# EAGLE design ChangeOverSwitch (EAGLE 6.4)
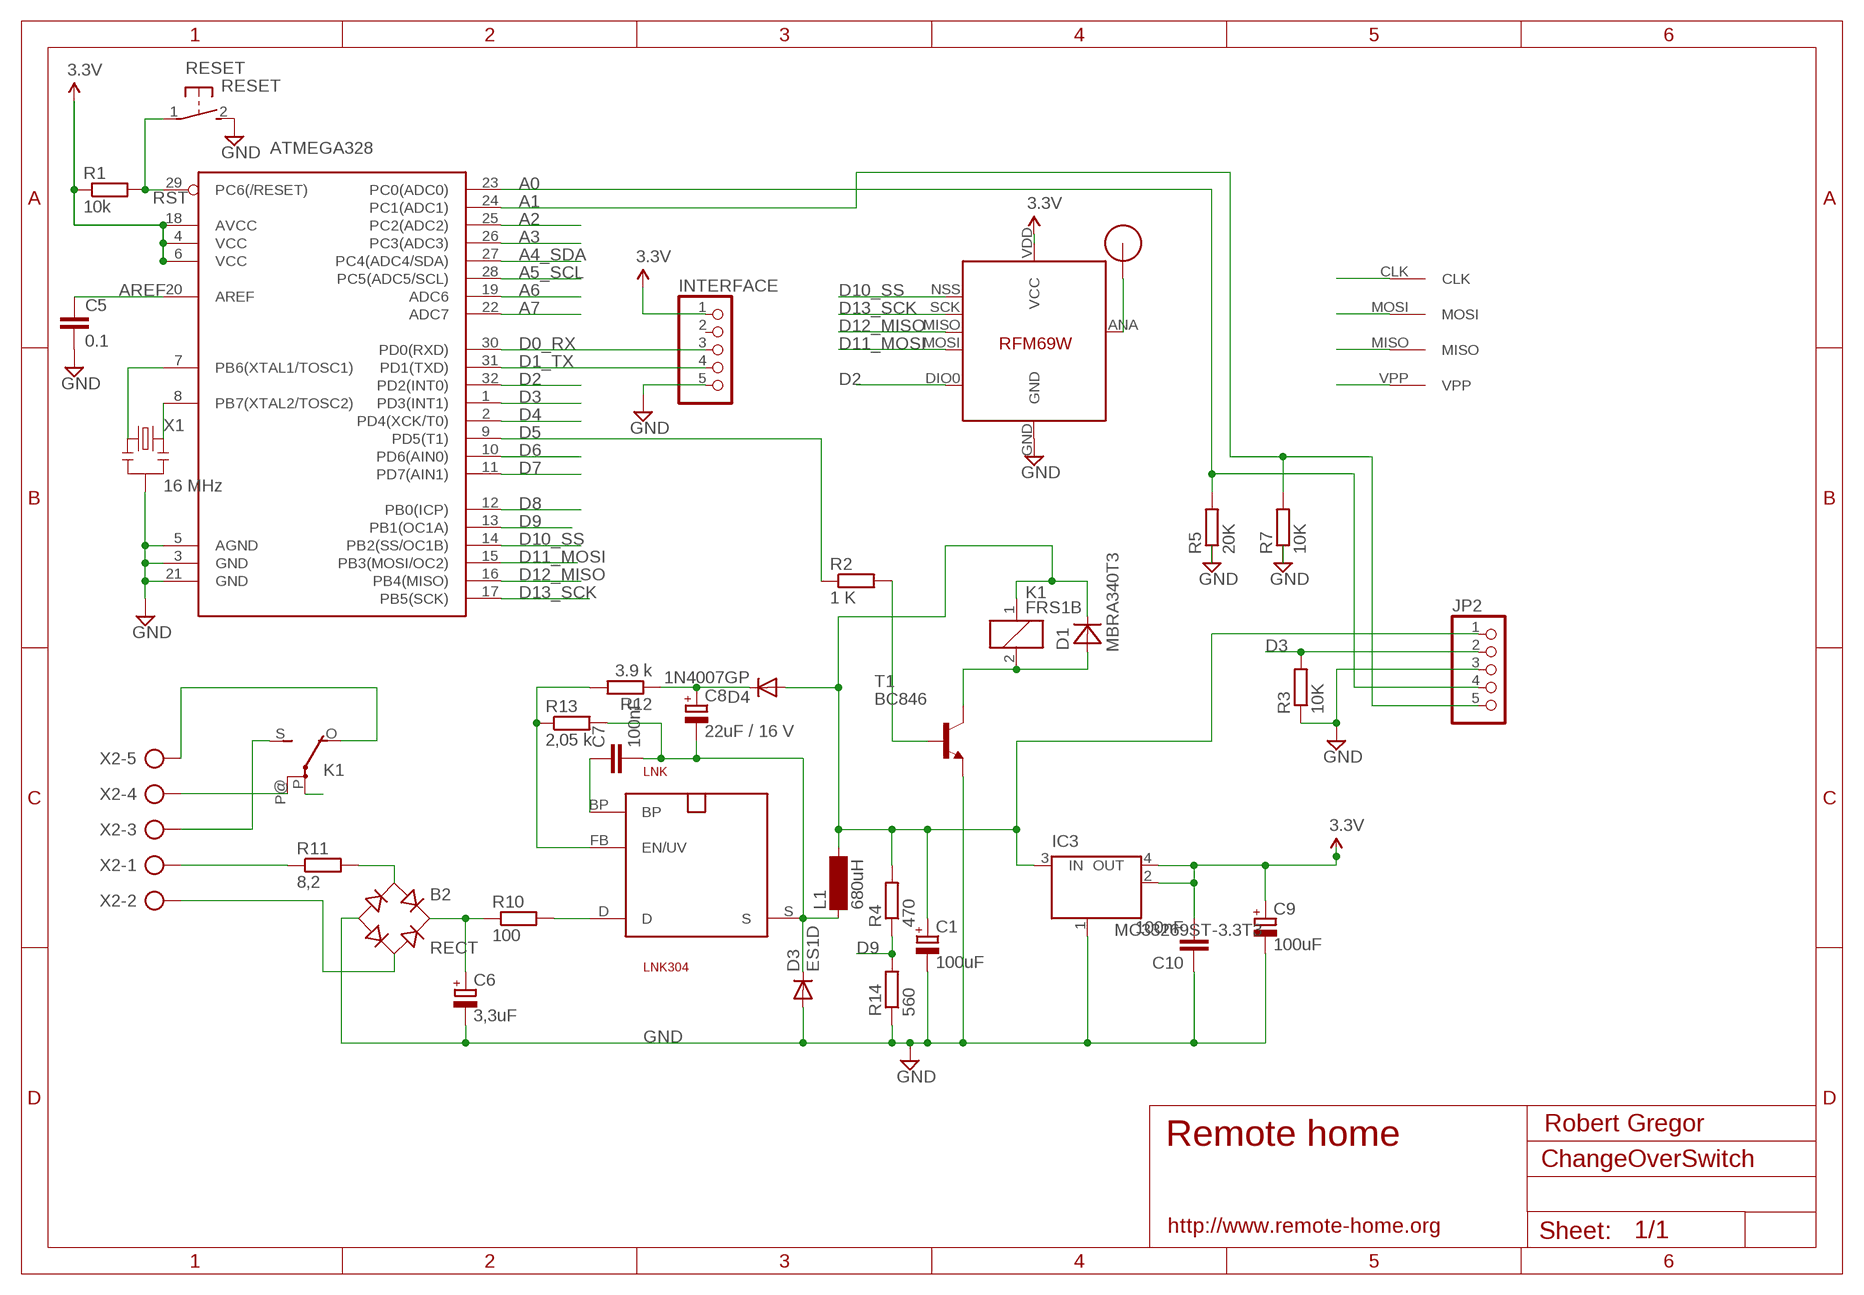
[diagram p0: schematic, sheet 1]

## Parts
ATMEGA328  ATMega-328  ATMEGA168/328TQFP32  [TQFP32-08]
B2  RECT  RECTIFIER-S40  [TO-269AA]
C1  100uF  CPOL-EUSMCB  [SMC_B]
C5  0.1  C-EUC2012  [C2012]
C6  3,3uF  CPOL-EUE5-10.5  [E5-10,5]
C7  100nF  C-EUC2012  [C2012]
C8  22uF / 16 V  CPOL-EUSMCC  [SMC_C]
C9  100uF  CPOL-EUSMCB  [SMC_B]
C10  100nF  C-EUC2012  [C2012]
D1  MBRA340T3  [SMA]
D3  ES1D  DIODE-DO214AC  [DO214AC]
D4  1N4007GP  DIODE-DO214AA  [DO214AA]
IC3  MC33269ST-3.3T3  [SOT223]
INTERFACE  PINHD-1X05_2.54-S  [1X05-S]
JP2  PINHD-1X05_2.00  [1X05M]
K1  FRS1B  [FRS1B]
L1  680uH  BS11  [BS11]
LNK  LNK304  SO-8C  [SO-8C]
R1  10k  R-EU_R2012  [R2012]
R2  1 K  R-EU_M2012  [M2012]
R3  10K  R-EU_M2012  [M2012]
R4  470  R-EU_M2012  [M2012]
R5  20K  R-EU_M2012  [M2012]
R7  10K  R-EU_M2012  [M2012]
R10  100  R-EU_R2512W  [R2512W]
R11  8,2  R-EU_0411/12  [0411/12]
R12  3.9 k  R-EU_M2012  [M2012]
R13  2,05 k  R-EU_M2012  [M2012]
R14  560  R-EU_M2012  [M2012]
RESET  RESET  DTSM-3  [DTSM-3]
RFM69  RFM69  [RFM69W-MINPADS]
T1  BC846  [SOT23]
U$1  RFM12B_ANTENNA  [RFM12B-ANTENNA]
U$2  AVRHEADERDIP  [AVRHEADER]
X1  16 MHz  RESONATORSMD  [RESONATOR-SMD]
X2  AK500/5  [AK500/5]

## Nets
5V: C1.+ D1.C D4.A IC3.3(IN) JP2.1 K1.1 L1.2 R4.2
A0: ATMEGA328.23(PC0(ADC0)) JP2.4 R5.2
A1: ATMEGA328.24(PC1(ADC1)) JP2.5 R7.2
A2: ATMEGA328.25(PC2(ADC2))
A3: ATMEGA328.26(PC3(ADC3))
A4_SDA: ATMEGA328.27(PC4(ADC4/SDA))
A5_SCL: ATMEGA328.28(PC5(ADC5/SCL))
A6: ATMEGA328.19(ADC6)
A7: ATMEGA328.22(ADC7)
AREF: ATMEGA328.20(AREF) C5.1
D0_RX: ATMEGA328.30(PD0(RXD)) INTERFACE.3
D1_TX: ATMEGA328.31(PD1(TXD)) INTERFACE.4
D2: ATMEGA328.32(PD2(INT0)) RFM69.DIO0
D3: ATMEGA328.1(PD3(INT1)) JP2.2 R3.2
D4: ATMEGA328.2(PD4(XCK/T0))
D5: ATMEGA328.9(PD5(T1)) R2.1
D6: ATMEGA328.10(PD6(AIN0))
D7: ATMEGA328.11(PD7(AIN1))
D8: ATMEGA328.12(PB0(ICP))
D9: ATMEGA328.13(PB1(OC1A)) R4.1 R14.2
D10_SS: ATMEGA328.14(PB2(SS/OC1B)) RFM69.NSS(SEL)
D11_MOSI: ATMEGA328.15(PB3(MOSI/OC2)) RFM69.MOSI U$2.MOSI
D12_MISO: ATMEGA328.16(PB4(MISO)) RFM69.MISO U$2.MISO
D13_SCK: ATMEGA328.17(PB5(SCK)) RFM69.SCK U$2.CLK
FB: LNK.FB(EN/UV) R12.2 R13.1
GND [power]: ATMEGA328.3(GND) ATMEGA328.5(AGND) ATMEGA328.21(GND) B2.- C1.- C5.2 C6.- C9.- C10.1 D3.A IC3.1(GND/ADJ) INTERFACE.5 JP2.3 R3.1 R5.1 R7.1 R14.1 RESET.2 RFM69.GND T1.2(E) X1.2
N$1: ATMEGA328.7(PB6(XTAL1/TOSC1)) X1.1
N$2: R2.2 T1.1(B)
N$3: RFM69.ANA(ANT) U$1.P$1
N$5: D1.A K1.2 T1.3(C)
N$6 [220V]: K1.P(2:P)
N$7 [220V]: R11.1 X2.1
N$8 [220V]: K1.P@(2:P) X2.4
N$9 [220V]: B2.AC2 X2.2
N$10: C7.2 C8.- D3.C L1.1 LNK.S R13.2
N$11 [220V]: K1.S(2:S) X2.3
N$12 [220V]: K1.O(2:O) X2.5
N$13 [220V]: LNK.D R10.2
N$14 [220V]: B2.+ C6.+ R10.1
N$15 [220V]: B2.AC1 R11.2
N$18: C7.1 LNK.BP
N$20: C8.+ D4.C R12.1
N$21: ATMEGA328.8(PB7(XTAL2/TOSC2)) X1.3
RST: ATMEGA328.29(PC6(/RESET)) R1.2 RESET.1 U$2.VPP
VCC: ATMEGA328.4(VCC) ATMEGA328.6(VCC) ATMEGA328.18(AVCC) C9.+ C10.2 IC3.2(OUT) IC3.4(OUT) INTERFACE.1 R1.1 RFM69.VDD(VCC) ; supply symbol labelled 3.3V
Unconnected: INTERFACE.2

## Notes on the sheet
- Robert Gregor
- Remote home
- http://www.remote-home.org

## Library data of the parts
ATMEGA328 = LowPowerLab:ATMEGA168/328: Atmel 32-pin 8-bit micro, 16k flash.
B2 = rectifier:RECTIFIER-: Rectifier
C1 C6 C8 C9 = resistor:CPOL-EU: POLARIZED CAPACITOR, European symbol
C5 C7 C10 = resistor:C-EU: CAPACITOR, European symbol
D1 = diode:MBRA340T3: Surface Mount Schottky Power Rectifier
D3 D4 = diode:DIODE-: DIODE
IC3 = linear:MC33269ST*: Adjustable Output Low Dropout Voltage Regulator 800 mA Source: http://www.onsemi.com/pub/Collateral/MC33269-D.PDF
INTERFACE JP2 = pinhead-2:PINHD-1X05: PIN HEADER
K1 = relay:FRS1B: RELAY 1 x switch, same as V23101-D6-A201, Siemens; OC_FARNELL: unknown; OC_NEWARK: unknown
L1 = inductor-neosid:BS: INDUCTOR; OC_FARNELL: unknown; OC_NEWARK: unknown
LNK = powerint:SO-8C: 700V MOSFET für Schaltnetz-Trafos. Pin 3 fehlt. SMD
R1-R5 R7 R10-R14 = resistor:R-EU_: RESISTOR, European symbol
RESET = switch-tact:DTSM-3
RFM69 = LowPowerLab:RFM69
T1 = transistor:BC846: NPN TRANSISTOR
U$1 = LowPowerLab:RFM12B_ANTENNA
U$2 = RemoteHome:AVRHEADER
X1 = SparkFun:RESONATOR: Resonator Small SMD resonator. This is the itty bitty 10/20MHz resonators with built in caps. CSTCE10M0G55 and CSTCE20M0V53. Footprint has been reviewed closely but hasn't been tested yet.
X2 = con-ptr500:AK500/5: CONNECTOR; OC_FARNELL: unknown; OC_NEWARK: unknown

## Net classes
1 power: width 0.381 mm, clearance 0.254 mm
2 220V: width 0.381 mm, clearance 0.508 mm

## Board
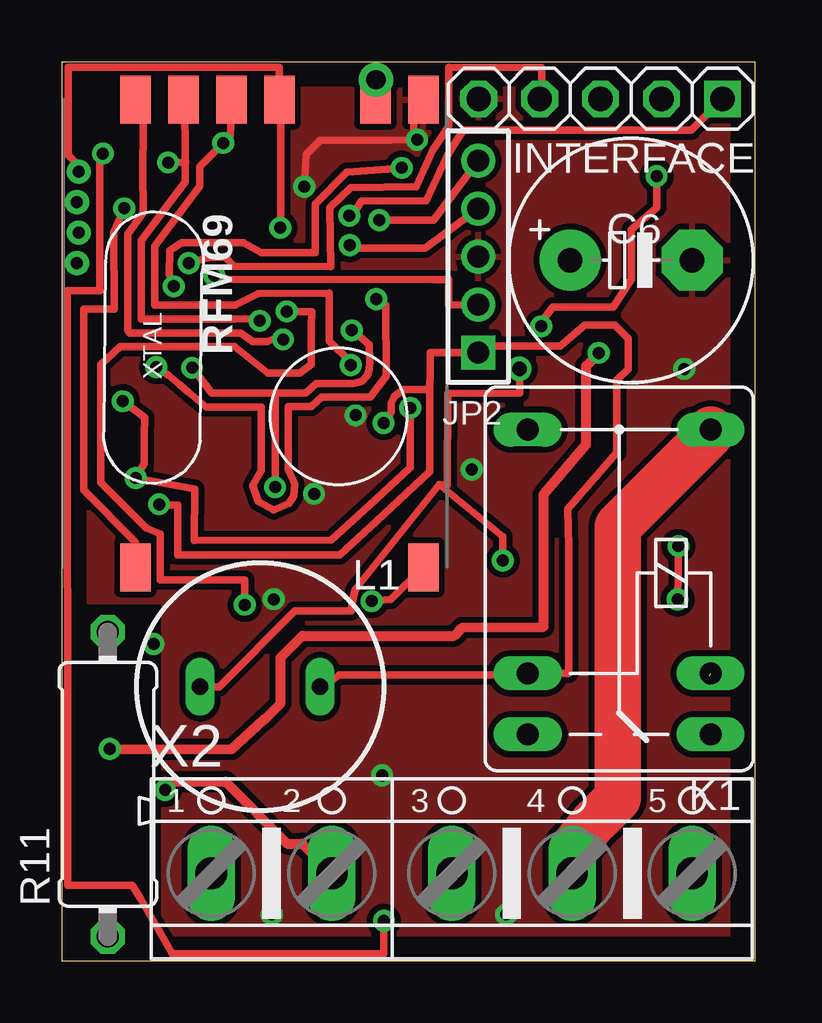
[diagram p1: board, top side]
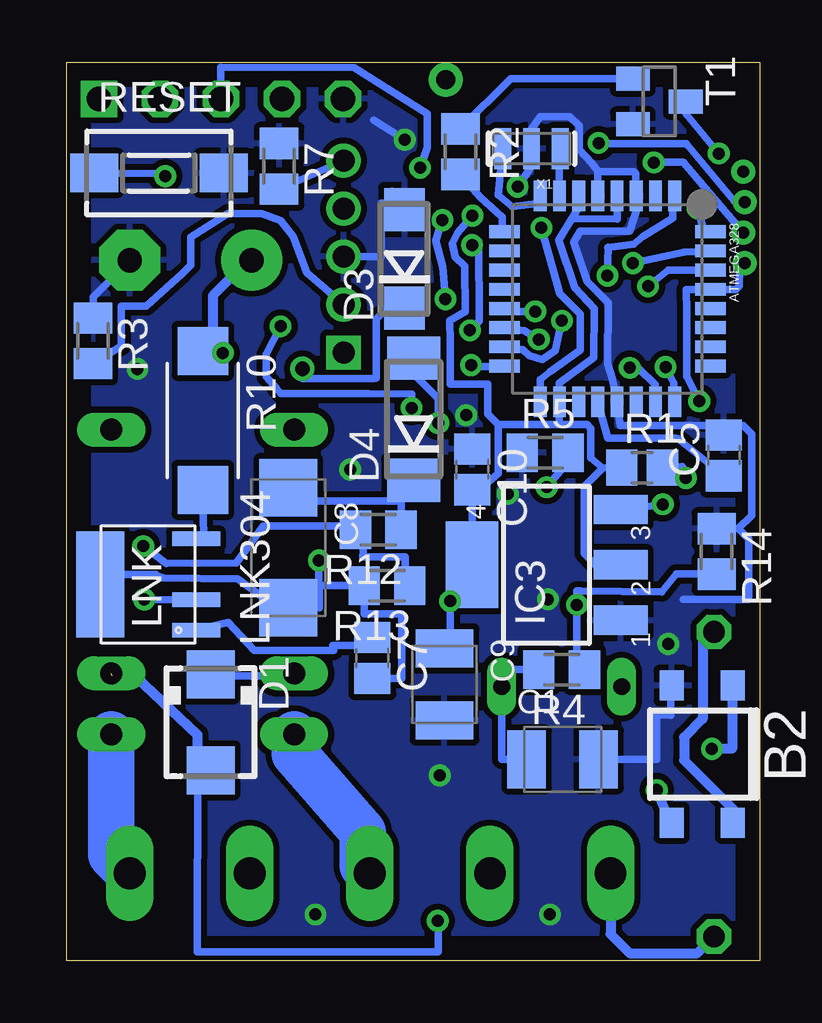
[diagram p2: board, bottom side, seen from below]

Size 28.88 x 37.45 mm. Coordinates in mm from the lower left corner, seen from the top.
Outline: 0,0 28.88,0 28.88,37.45 0,37.45 0,0
Copper layers (1*16): Top 0.035mm / dielectric 1.5mm / Bottom 0.035mm
Design rules "default": minimum track width 10mil, minimum drill 24mil, track to track 8mil, track to pad 8mil, pad to pad 8mil, via to via 8mil, smd to smd 8mil, copper to edge 40mil, drill to drill 8mil, minimum pad ring 10mil, minimum via ring 8mil, stop-mask expansion 4mil, vias tented up to drill 0mil, thermal gap 10mil

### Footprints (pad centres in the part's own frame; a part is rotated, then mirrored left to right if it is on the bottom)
TQFP32-08 = smd 1.27 x 0.533: 1 -4.293,2.8; 2 -4.293,2; 3 -4.293,1.2; 4 -4.293,0.4; 5 -4.293,-0.4; 6 -4.293,-1.2; 7 -4.293,-2; 8 -4.293,-2.8; 17 4.293,-2.8; 18 4.293,-2; 19 4.293,-1.2; 20 4.293,-0.4; 21 4.293,0.4; 22 4.293,1.2; 23 4.293,2; 24 4.293,2.8 | smd 0.533 x 1.27: 9 -2.8,-4.293; 10 -2,-4.293; 11 -1.2,-4.293; 12 -0.4,-4.293; 13 0.4,-4.293; 14 1.2,-4.293; 15 2,-4.293; 16 2.8,-4.293; 25 2.8,4.293; 26 2,4.293; 27 1.2,4.293; 28 0.4,4.293; 29 -0.4,4.293; 30 -1.2,4.293; 31 -2,4.293; 32 -2.8,4.293
TO-269AA = smd 1 x 1.25: + -1.28,-2.855; - 1.28,-2.855; AC1 -1.28,2.855; AC2 1.28,2.855
SMC_B = smd 1.6 x 2.4: + -1.5,0; - 1.5,0
C2012 = smd 1.3 x 1.5: 1 -0.85,0; 2 0.85,0
E5-10,5 = drill 1.016 pad 2.54: + -2.54,0 | drill 1.016 pad 2.54 octagon: - 2.54,0
SMC_C = smd 2.4 x 2.4: + -2.5,0; - 2.5,0
SMA = smd 2 x 2: A 2,0; C -2,0
DO214AC = smd 1.8 x 1.7: A 2.05,0; C -2.05,0
DO214AA = smd 1.8 x 2.2: A 2.55,0; C -2.55,0
SOT223 = smd 1.219 x 2.235: 1 -2.311,-3.099; 2 0,-3.099; 3 2.311,-3.099 | smd 3.6 x 2.2: 4 0,3.099
1X05-S = drill 1.016 square: 1 -5.08,0 | drill 1.016 octagon: 2 -2.54,0; 3 0,0; 4 2.54,0; 5 5.08,0
1X05M = drill 0.914 square: 1 -4,0 | drill 0.914: 2 -2,0; 3 0,0; 4 2,0; 5 4,0
FRS1B = drill 0.914 long: 1 0,3.81; 2 0,-3.81; O -2.54,-3.81; P 10.16,3.81; P@ 10.16,-3.81; S -2.54,3.81
BS11 = drill 0.7 long: 1 -2.5,0; 2 2.5,0
SO-8C = smd 0.6 x 2: BP -1.905,-2; D 1.905,-2; FB -0.635,-2 | smd 4.41 x 2: S 0,2
R2012 = smd 1.3 x 1.5: 1 -0.85,0; 2 0.85,0
M2012 = smd 1.3 x 1.6: 1 -0.95,0; 2 0.95,0
R2512W = smd 2 x 2.1: 1 -2.896,0; 2 2.896,0
0411/12 = drill 0.914 octagon: 1 -6.35,0; 2 6.35,0
DTSM-3 = smd 2 x 1.6: 1 -2.7,0; 2 2.7,0
RFM69W-MINPADS = smd 2 x 1.27: ANA 8,-5; DIO0 -11.5,5; GND 8,-7; MISO 8,1; MOSI 8,3; NSS 8,5; SCK 8,-1; VDD -11.5,-7
SOT23 = smd 1 x 1.4: 1 -0.95,-1.1; 2 0.95,-1.1; 3 0,1.1
RFM12B-ANTENNA = drill 0.8 pad 1.422: P$1 0,0
AVRHEADER = drill 0.5: CLK 2.54,0; MISO 1.27,0.07; MOSI 0,0; VPP -1.27,0.072
RESONATOR-SMD = smd 0.7 x 1.7: 1 -1.2,0; 2 0,0; 3 1.2,0
AK500/5 = drill 1.321 long: 1 -10.033,0; 2 -5.004,0; 3 0,0; 4 5.004,0; 5 10.008,0

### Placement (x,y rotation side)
ATMEGA328  6.35,27.59 270 bottom
B2  2.4,8.62 180 bottom
C1  8.22,8.4 0 bottom
C5  1.5,21.07 90 bottom
C6  23.71,29.21 0 top
C7  16.15,12.63 270 bottom
C8  19.65,17.22 270 bottom
C9  13.14,11.52 270 bottom
C10  11.98,20.49 270 bottom
D1  22.89,9.95 270 bottom
D3  14.8,29.26 90 bottom
D4  14.42,22.58 90 bottom
IC3  8.89,16.51 90 bottom
INTERFACE  22.45,35.94 180 top
JP2  17.34,29.36 90 top
K1  23.22,11.99 90 top
L1  8.26,11.43 0 top
LNK  25.49,15.69 90 bottom
R1  4.91,20.57 0 bottom
R2  12.47,33.74 90 bottom
R3  27.79,25.85 270 bottom
R4  8.26,12.14 180 bottom
R5  8.94,21.18 0 bottom
R7  20.03,33.13 270 bottom
R10  23.21,22.53 270 bottom
R11  1.91,7.36 90 top
R12  15.9,17.98 180 bottom
R13  15.53,15.64 180 bottom
R14  1.8,17.07 270 bottom
RESET  25.04,32.85 0 bottom
RFM69  8.06,27.91 90 top
T1  4.19,35.83 270 bottom
U$1  13.08,36.73 0 top
U$2  0.69,30.36 90 top
X1  9.51,33.86 180 bottom
X2  16.25,3.65 0 top

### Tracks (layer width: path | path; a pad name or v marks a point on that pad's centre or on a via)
5V  (via drill 0.5)
  Top 0.305: L1.2 10.88,11.43 10.89,11.44 10.89,11.38 11.56,11.92 18.64,11.93 18.87,11.92 K1.1 19.68,11.97 21.12,11.97 21.12,17.23 21.08,18.85 23.12,21.19 23.12,24.21 23.59,24.68 23.59,25.95 23.02,26.51 21.78,26.51 20.76,25.62 17.73,25.62 JP2.1 16.34,25.37 15.9,25.36 15.35,25.36 15.35,24.29 15.33,24.14 | 15.33,24.14 15.31,20.39 13.09,18.31 11.56,16.91 4.82,16.91 4.82,17.62 4.82,19.01 4.4,19.01 v4.04,19.03 | v13.4,22.42 13.73,22.88 13.72,23.26 13.85,23.53 14.21,23.81 15.33,23.81 15.33,24.14
  Bottom 0.305: D1.C 22.82,11.88 19.51,11.88 K1.1 | 5.68,18.93 IC3.3 | IC3.3 5.43,18.82 | v4.04,19.03 5.77,18.8 IC3.3 | R4.2 10.76,12.14 L1.2 10.76,8.4 C1.+ | D4.A 14.42,24.46 13.4,23.43 v13.4,22.42
A0  (via drill 0.5)
  Top 0.305: JP2.4 15.94,30.31 15.13,29.72 12.04,29.72 v11.99,29.84 | v12.08,26.29 12.15,26.26 12.81,25.69 12.82,24.96 12.8,24.64 12.71,24.39 12.5,24.17 12.39,24.13 12.12,24.06 10.6,24.07 10.15,23.68 9.13,23.68 | 9.13,23.68 6.25,23.68 v5.42,24.73 | v8.88,19.75 8.88,23.68 9.13,23.68
  Bottom 0.305: v11.99,29.84 12.02,30 11.71,30 11.69,26.68 v12.08,26.29 | v5.42,24.73 5.03,24.7 4.35,24.02 ATMEGA328.23 | R5.2 7.94,20.87 v8.88,19.75
A1  (via drill 0.5)
  Top 0.305: JP2.5 15.5,30.89 v13.22,30.88 | v3.92,24.75 4.43,24.43 4.92,24.01 5.25,23.72 6.01,23.09 8.3,23.09 8.3,20.43 7.94,19.82 8.18,19.15 8.83,18.8 9.44,19.06 9.66,19.38 9.7,19.87 9.42,20.49 9.42,23.11 10.38,23.11 10.82,23.51 12.84,23.51 13.51,24.37 13.49,27.34 v13.1,27.59
  Bottom 0.305: v13.22,30.88 13.51,30.02 13.21,28.93 13.13,27.99 v13.1,27.59 | ATMEGA328.24 3.58,24.08 v3.92,24.75 | R7.2 JP2.5
AREF
  Bottom 0.305: 6.77,23.03 ATMEGA328.20 6.33,21.79 3.52,21.79 3.43,21.78 C5.1
D0_RX  (via drill 0.5)
  Top 0.305: v4.66,28.12 4.48,28.58 4.48,29.61 4.99,29.95 7.56,29.94 8.3,29.53 10.54,29.53 10.54,31.55 11.87,32.88 13.57,33.01 v14.15,33.06
  Bottom 0.305: ATMEGA328.30 3.81,28.79 v4.66,28.12 | v14.15,33.06 13.85,33.9 13.85,35.32 16.91,37.23 22.45,37.25 INTERFACE.3
D1_TX  (via drill 0.5)
  Top 0.305: INTERFACE.4 19.99,36.15 19.98,37.24 16.11,37.25 16.11,34.79 15.45,33.8 14.76,32.27 12.03,32.24 11.16,31.39 11.2,28.94 7.16,28.95 6.81,29.33 6.45,29.33 6.14,29.33 6.01,29.29 v5.29,29.09
  Bottom 0.305: ATMEGA328.31 3.15,29.55 v5.29,29.09
D2  (via drill 0.5)
  Top 0.305: v2.6,31.37 2.16,30.4 2.17,27.18 0.9,27.18 0.91,19.63 3.06,17.46 RFM69.DIO0 3.08,16.42
  Bottom 0.305: v2.6,31.37 2.33,30.45 2.1,30.37 2.08,30.39 ATMEGA328.32
D3  (via drill 0.5)
  Top 0.305: JP2.2 16.11,27.34 16.11,28.29 16.12,28.4 15.49,28.41 6.69,28.42 v6.35,28.57
  Bottom 0.305: v6.35,28.57 6.31,29.76 6.33,29.74 5.26,29.87 4.87,30.19 3.62,30.97 3.62,31.26 3.62,31.81 ATMEGA328.1 | R3.2 26.61,25.62 26.61,27.16 26.61,27.3 25.56,27.3 24.09,28.63 23.72,29 23.72,30.17 23.71,30.17 22.17,31.16 20.75,31.16 19.96,30.85 19.43,30.2 18.89,28.68 JP2.2
D5
  Bottom 0.305: ATMEGA328.9 10.74,30.39 10.72,31 11.64,31.84 R2.1
D9  (via drill 0.5)
  Top 0.305: v9.36,27.07 10.4,27.07 10.39,26.44 10.39,24.85 9.91,24.51 8.56,24.51 7.19,25.61 2.42,25.61 1.62,24.85 1.62,19.94 3.5,18.04 4.09,17.8 4.09,15.88 7.61,15.87 v7.62,14.84
  Bottom 0.305: ATMEGA328.13 10.39,27.07 v9.36,27.07 | R14.2 1.76,16.12 1.75,16.12 3.48,16.12 4.09,15.38 7.45,15.42 7.62,15.42 7.62,15.33 v7.62,14.84 7.62,13.01 7.62,12.16 7.44,12.16 7.67,12.14 R4.1
D10_SS  (via drill 0.5)
  Top 0.305: RFM69.NSS 3.39,34.92 3.37,32.69 3.39,31.5 3.39,31.19 2.73,30.3 2.73,26.3 2.83,26.18 7.45,26.18 7.95,25.82 8.55,25.82 9.11,26.06 v9.21,25.91
  Bottom 0.305: ATMEGA328.14 10.62,26.37 9.82,26.28 v9.21,25.91
D11_MOSI  (via drill 0.5)
  Top 0.305: v8.24,26.68 8.08,26.77 7.21,26.76 6.18,26.76 3.29,26.76 3.29,30.04 5.13,32.49 5.14,33.39 | 5.14,33.39 5.13,35.87 RFM69.MOSI | v4.42,33.28 5.16,33.29 5.14,33.39
  Bottom 0.305: ATMEGA328.15 9.88,25.48 9.61,25.24 9.06,25.07 8.52,25.45 v8.24,26.68 | U$2.MOSI 1.9,31.78 3.18,33.29 4.54,33.29 v4.42,33.28
D12_MISO  (via drill 0.5)
  Top 0.305: RFM69.MISO 7.04,34.81 7.02,34.4 6.94,34.28 6.59,33.93 v6.72,34.1 5.74,33.1 5.74,32.29 3.87,29.8 3.87,27.85 3.87,27.34 7.21,27.34 8.17,27.82 11.14,27.83 11.14,25.85 12.03,24.96 v12.03,24.84
  Bottom 0.305: v12.03,24.84 12.04,24.77 11.46,24.77 10.51,24.77 ATMEGA328.16 | v6.72,34.1 6.68,34.06 3.07,34.06 1.06,31.66 0.83,31.63 U$2.MISO
D13_SCK  (via drill 0.5)
  Top 0.305: v9.1,30.56 9.12,30.65 9.12,34.62 9.12,35.87 RFM69.SCK | 9.26,36.1 RFM69.SCK | U$2.CLK 0.55,33.29 0.25,33.58 0.27,33.58 0.27,37.25 9.06,37.25 RFM69.SCK
  Bottom 0.305: ATMEGA328.17 9.15,24.23 8.74,24.57 7.49,25.46 7.47,26.97 8.33,27.81 v9.1,30.56
FB  (via drill 0.5)
  Top 0.305: v25.69,17.29 25.69,16.2 v25.65,15.07
  Bottom 0.305: v25.69,17.29 24.73,16.57 21.81,16.6 20.68,18.14 17.64,18.14 16.98,18.16 R12.2 16.66,17.91 16.51,17.31 16.54,16.85 14.77,16.83 14.8,15.29 R13.1 | v25.65,15.07 23.5,15.04 LNK.FB
GND  (via drill 0.5)
  Top 0.305: RFM69.GND 14.59,35.86 14.65,35.46 14.65,34.39 v14.79,34.24 13.7,34.2 10.75,34.21 10.18,33.63 v10.09,32.28
  Bottom 0.305: ATMEGA328.5 6.75,32.88 6.73,32.9 | 6.73,32.9 5.25,32.9 5.17,32.82 5.17,31.62 ATMEGA328.3 5.07,31.52 5.42,30.42 7.49,30.42 7.67,30.1 7.76,29.96 7.19,28.31 6.31,27.44 6.34,24.89 6.15,24.28 ATMEGA328.21 5.97,23.3 5.81,22.31 1.88,22.31 | 6.73,32.9 7,33.26 7.52,33.82 7.52,34.82 7.91,35.18 9.15,35.18 9.51,34.66 X1.2 9.51,33.12 v10.09,32.28 | D3.A 15.16,31.93 | 15.16,31.93 15.32,32.08 | 14.4,30.86 14.71,31.54 D3.A | R3.1 27.77,27.66 C6.- | 1.88,22.31 C5.2 | R14.1 0.89,18.02 | 0.89,18.02 0.46,17.59 0.46,15.25 0.47,15.06 1.09,15.06 3.18,15.07 | 1.88,22.31 0.7,22.31 0.34,21.95 0.34,18.57 0.89,18.02 | D3.A 14.82,31.82 | JP2.3 15.78,29.36 15.77,31.59 15.5,31.59 15.16,31.93 | C1.- 4.29,8.4 4.29,10.25 3.72,10.25 | 3.72,10.25 3.72,10.24 | 16.08,35.05 v14.79,34.24 | B2.- 3.72,11.47 3.72,10.25
  Bottom 0.406: R3.1 27.74,27.02
  other vias: 12.23,22.74 13.34,7.73 3.82,13.21 18.52,1.93 8.74,1.94 10.5,19.47 8.83,15.07 17.07,20.48 25.93,24.68
  pour Top: 0.13,37.3 28.75,37.3 28.75,0.13 4.26,0.13 4.26,14.99 0.18,14.96 0.13,37.23
  pour Bottom: 0.19,37.3 28.75,37.3 28.75,0.13 0.16,0.13 0.16,37.33
N$1
  Bottom 0.305: ATMEGA328.7 8.35,33.48 X1.1
N$2
  Bottom 0.305: T1.1 10.38,36.78 R2.2
N$3
  Top 0.406: RFM69.ANA 13.12,35.87 U$1.P$1
N$5  (via drill 0.5)  (1 unrouted)
  Top 0.305: v13.41,1.67 | v13.41,1.67 13.41,0.3 4.6,0.3 3.28,2.58 2.92,3.15 0.23,3.15 0.22,27.94 1.59,27.94 1.58,28.01 1.57,33.11 1.6,33.37 v1.71,33.66
  Bottom 0.305: D1.A 22.86,8.15 23.42,8.15 23.45,0.37 13.39,0.37 13.39,1.29 v13.41,1.67 | T1.3 3.06,35.29 v1.71,33.66
  Bottom 0.406: 26.98,11.88 26.03,11.86 23.44,9.42 23.44,8.74 D1.A
N$7
  Bottom 0.406: X2.1 6.22,1.11 5.43,0.33 2.6,0.33 R11.1
N$8
  Top 1.93: K1.P@ 27.02,21.98 23.15,18.1 23.15,6.78 22.23,5.86 22.16,5.79 21.26,4.67 21.26,3.68 X2.4
N$9  (via drill 0.5)
  Top 0.406: v4.29,7.12 4.35,7.43 4.3,7.48 6.82,7.46 9.39,4.89 10.01,4.89 X2.2
  Bottom 0.406: B2.AC2 3.68,5.62 v4.29,7.12
N$10  (via drill 0.5, 0.6)
  Top 0.305: v19.06,24.68 19.06,23.66 16.06,23.65 16.06,19.85 15.71,19.85 | 15.71,19.85 12.22,15.49 12.07,14.85 12.06,14.58 9.71,14.58 6.55,11.43 L1.1 | v18.37,16.7 18.37,17.7 15.71,19.85
  Bottom 0.305: LNK.S 26.88,16.1 25.18,16.12 25.28,16.11 24.86,15.95 21.76,15.92 20,14.64 C8.- | C8.- 18.73,15.65 R13.2 | R13.2 16.47,15.19 | D3.C 14.76,27.3 14.82,27.25 15.49,27.25 15.99,26.75 15.99,24.29 16.09,24.28 19.06,24.28 v19.06,24.68 | C7.2 14.91,11.78 14.91,14.46 16.48,14.46 R13.2 | v18.37,16.7 18.36,14.72 C8.-
N$11
  Bottom 1.93: K1.S 19.39,8.62 16.55,5.37 16.55,3.96 X2.3
N$12
  Bottom 1.93: K1.O 27.02,4.42 X2.5
N$13
  Bottom 0.305: R10.2 23.17,17.59 LNK.D
N$14  (via drill 0.5)
  Top 0.406: v2,8.84 7.07,8.83 8.41,10.05 8.42,10.05 9.11,10.74 9.11,12.65 10.02,13.55 16.34,13.55 16.68,13.9 20.06,13.93 20.07,19.43 21.84,21.52 21.84,24.15 | 21.84,24.15 | 21.84,24.15 21.84,24.8 v22.37,25.35
  Bottom 0.305: R10.1 22.45,25.43 v22.37,25.35 | B2.+ 1.15,11.47
  Bottom 0.406: C6.+ 21.31,29.21 22.79,27.73 22.79,25.82 R10.1 | v2,8.84 1.15,8.84 1.15,11.47
N$15
  Bottom 0.406: R11.2 2.38,13.71 2.38,10.08 2.4,10.08 3.15,9.32 3.15,8.37 1.12,6.33 B2.AC1 | B2.AC1
N$18
  Bottom 0.305: LNK.BP 22.16,14.1 21.07,12.94 17.76,12.95 17.79,13.15 15.73,13.15 C7.1
N$20
  Bottom 0.305: R12.1 14.95,19.38 D4.C 14.96,20.17 14.96,19.17 18.61,19.17 18.61,19.27 C8.+
N$21
  Bottom 0.305: X1.3 10.9,31.93 10.31,31.43 9.15,31.6 ATMEGA328.8
RST  (via drill 0.5)
  Top 0.305: v24.78,32.71 24.78,31.41 23.71,30.49 23.71,28.41 22.97,27.25 22.53,27.25 20.45,27.25 19.97,26.63 v19.97,26.45 | v14.51,23.05 14.51,20.57 12.81,18.98 11.21,17.54 5.52,17.53 5.53,19.68 v3.08,20.12 3.44,20.74 3.44,21.91 3.44,22.66 v2.53,23.33
  Bottom 0.305: RESET.1 24.73,32.82 v24.78,32.71 | v14.51,23.05 14.51,23.63 16.31,23.64 17.16,23.66 19.28,23.66 19.96,23.65 20.16,23.89 20.56,24.36 20.56,25.29 v19.97,26.45 | R1.2 3.23,20.61 v3.08,20.12 | U$2.VPP 0.83,29.09 0.84,28.79 0.85,28.14 1,27.99 ATMEGA328.29 | ATMEGA328.29 | ATMEGA328.29 3.06,27.99 3.05,27.05 3.05,24.36 v2.53,23.33
VCC  (via drill 0.5)
  Top 0.305: RFM69.VDD 13.71,15.06 v12.91,14.99 | v11.97,31.07 12.16,31.16 12.47,31.67 15.19,31.69 16.04,33.52 16.32,34 16.72,34.62 17.78,34.62 26.21,34.62 INTERFACE.1
  Bottom 0.305: IC3.2 | 8.37,30.04 7.72,28.06 6.9,27.19 6.92,25.14 8.35,24.09 ATMEGA328.18 8.35,22.35 | 8.37,30.04 7.52,31.44 ATMEGA328.6 | ATMEGA328.4 5.95,30.93 7.84,30.95 8.37,30.04 | v11.97,31.07 12.59,30.35 12.82,29.91 12.7,29.35 12.29,28.97 12.27,27.06 12.92,26.68 12.9,25.82 12.9,25.35 12.89,24.04 11.34,24.05 11.34,23.68 11.33,22.8 11.26,22.71 10.9,22.35 | R1.1 6.55,20.55 | IC3.2 | v12.91,14.99 13.1,14.99 | v12.91,14.99 IC3.4 | 12.02,16.42 12.02,16.51 IC3.4 | C9.+ 12.91,13.07 v12.91,14.99 | 10.9,22.35 10.9,20.31 11.34,19.93 11.69,19.76 C10.2 11.99,19.82 IC3.4 | 10.9,22.35 8.35,22.35 | 8.35,22.35 7.18,22.35 7.04,22.19 7.04,20.97 6.55,20.55 | IC3.2 6.86,16.51 7.33,16.98 7.33,19.78 6.55,20.55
